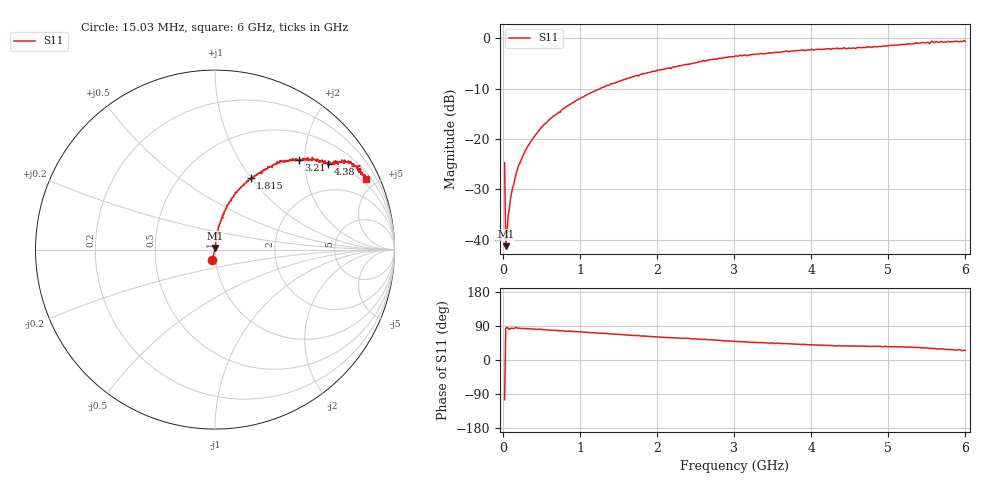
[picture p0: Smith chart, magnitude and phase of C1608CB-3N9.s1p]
!	Network	Analyzer	HP8753E.07.74:	Oct	30	2002	Serial	No.	JP38451487
!	Hewlett-Packard
!	7	Sep	2009	9:30:22
!	Frequency	S11
#	HZ	S	RI	R	50
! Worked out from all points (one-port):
!   400 points, 15.03 MHz to 6 GHz, reference 50 ohm
!   lowest |S11| = -41.3 dB at 30.03 MHz (marker M1), VSWR 1.02, Z = 50.1 + j0.858 ohm
!   |S11| at or under -10 dB: start of sweep to 1.259 GHz
!   S11 on the Smith chart (normalised r, x): 15.03 MHz: 0.96, -0.11; 1.815 GHz: 1.00, +0.99; 3.21 GHz: 1.00, +1.87; 4.38 GHz: 1.03, +2.62; 6 GHz: 0.75, +4.35
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1.502992e7  -0.015 -0.0561
3.002985e7  0.00103 0.00856
4.502978e7  0.000638 0.011
6.00297e7  0.0017 0.0168
9.002955e7  0.00264 0.0248
1.200294e8  0.0036 0.0328
1.95029e8  0.00549 0.0539
2.850286e8  0.00947 0.0767
4.950275e8  0.0202 0.13
7.650262e8  0.0423 0.192
1.110024e9  0.0833 0.268
1.515022e9  0.145 0.345
1.815021e9  0.199 0.397
2.265019e9  0.279 0.449
3.015015e9  0.432 0.508
3.210014e9  0.467 0.498
3.765011e9  0.547 0.502
4.380008e9  0.63 0.477
4.515007e9  0.636 0.472
5.265004e9  0.727 0.488
5.445003e9  0.772 0.474
5.520002e9  0.778 0.469
5.535002e9  0.752 0.453
5.565002e9  0.808 0.468
5.595002e9  0.775 0.462
5.625002e9  0.814 0.445
5.715001e9  0.795 0.442
6e9  0.841 0.396
